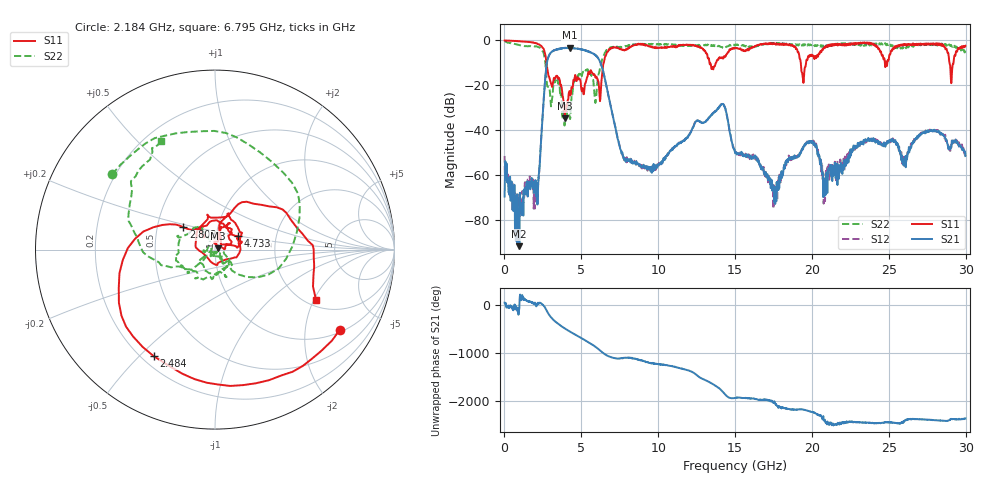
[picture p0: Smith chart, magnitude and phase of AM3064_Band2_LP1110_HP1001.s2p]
# Hz S DB R 50.0
!freq dBS11 angS11 dBS21 angS21 dBS12 angS12 dBS22 angS22
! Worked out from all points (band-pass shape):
!   1600 points, 10 MHz to 29.98 GHz, reference 50 ohm
!   highest |S21| = -3.26 dB at 4.246 GHz (marker M1); lowest = -91.7 dB at 965.9 MHz (marker M2)
!   |S21| within 3 dB of the highest: 2.933 GHz to 5.853 GHz (2.92 GHz wide, 66.5 % of centre)
!   lowest |S11| = -34.8 dB at 3.927 GHz (marker M3), VSWR 1.04, Z = 51.7 + j0.725 ohm
!   |S11| at or under -10 dB: 2.731 GHz to 6.453 GHz (3.722 GHz wide, 81 % of centre); 13.34 GHz to 13.75 GHz (414.6 MHz wide, 3.06 % of centre); 19.27 GHz to 19.61 GHz (340.9 MHz wide, 1.75 % of centre)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
!   |S22| runs from -37.9 to -0.2 dB; largest |S21 - S12| = 0.02
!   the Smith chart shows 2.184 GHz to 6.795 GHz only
!   S11 on the Smith chart (normalised r, x): 2.184 GHz: 1.09, -3.07; 2.484 GHz: 0.25, -0.55; 2.803 GHz: 0.68, +0.18; 4.733 GHz: 1.28, +0.20; 6.795 GHz: 2.22, -2.08
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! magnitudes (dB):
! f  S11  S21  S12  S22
! 10 MHz  0.0  -69.5  -51.5  -0.2
! 965.9 MHz  -0.3  -91.7  -69.7  -2.1
! 2.184 GHz  -1.7  -66.0  -64.0  -3.0
! 2.484 GHz  -3.3  -33.2  -33.3  -4.8
! 2.803 GHz  -13.3  -8.6  -8.6  -20.6
! 3.927 GHz  -34.8  -3.4  -3.3  -33.0
! 4.246 GHz  -22.7  -3.3  -3.4  -34.5
! 4.733 GHz  -16.4  -3.7  -3.6  -15.8
! 5.015 GHz  -22.1  -4.0  -3.9  -15.7
! 5.933 GHz  -16.7  -6.7  -6.7  -27.2
! 6.795 GHz  -4.0  -25.6  -25.6  -3.4
! 7.826 GHz  -4.4  -52.6  -52.3  -2.8
! 10 GHz  -3.3  -55.5  -55.7  -1.7
! 14.14 GHz  -7.7  -28.5  -28.5  -3.0
! 15 GHz  -3.2  -50.3  -49.4  -1.9
! 17.63 GHz  -1.7  -67.8  -67.6  -1.2
! 19.99 GHz  -6.4  -45.7  -45.6  -1.7
! 20.87 GHz  -2.7  -62.8  -64.0  -2.7
! 25 GHz  -8.6  -45.7  -44.7  -1.6
! 28.28 GHz  -1.4  -41.1  -41.1  -2.5
! 29.08 GHz  -17.8  -46.3  -46.3  -2.5
! 29.98 GHz  -2.4  -51.5  -51.5  -4.6
